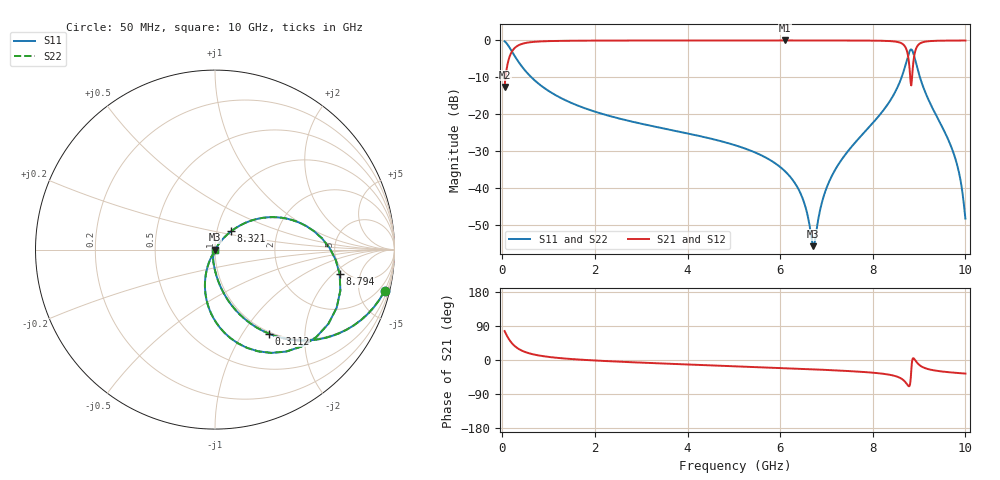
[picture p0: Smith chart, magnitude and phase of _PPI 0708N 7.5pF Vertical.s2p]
! S-Parameter data specifications (vertical orientation):
! Substrate: 40-mil Rogers 3003C, Substrate thickness, H=1.016mm, Dielectric constant, Er=3, Conductor thickness, T_mtl=0.043mm, Loss Tangent, Tand=0.003
! PCB Mounting Pad Footprint: Pad width, PadW=2.54mm , Pad length, PadL=0.51mm , Pad gap, PadG (edge-to-edge)=0.71mm , Reference planes=1.73mm apart
! Created Tue Jan 16 08:46:27 2018
# GHz S MA R 50
! 2 Port Network Data from SP1.SP block
! freq  magS11  angS11  magS21  angS21  magS12  angS12  magS22  angS22
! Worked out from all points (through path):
!   801 points, 50 MHz to 10 GHz, reference 50 ohm
!   highest |S21| = -0.02 dB at 6.107 GHz (marker M1); lowest = -12.6 dB at 50 MHz (marker M2)
!   group delay of S21, straight-line fit = 16 ps
!   lowest |S11| = -55.8 dB at 6.716 GHz (marker M3), VSWR 1.00, Z = 50.1 - j0.081 ohm
!   |S11| at or under -10 dB: 628.1 MHz to 8.622 GHz (7.994 GHz wide, 173 % of centre); 9.018 GHz to end of sweep
!   |S22| runs from -55.8 to -0.2 dB; largest |S21 - S12| = 0
!   S11 on the Smith chart (normalised r, x): 50 MHz: 0.97, -8.22; 311.2 MHz: 0.97, -1.32; 8.321 GHz: 1.17, +0.24; 8.794 GHz: 4.46, -2.45; 10 GHz: 1.00, -0.01
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0.05  0.9724 -13.7  0.2334 76.3  0.2334 76.3  0.9724 -13.7
0.1619375  0.7895 -38.5  0.6135 51.5  0.6135 51.5  0.7895 -38.5
0.3111875  0.5567 -57.3  0.8304 32.7  0.8304 32.7  0.5567 -57.3
0.7091875  0.2835 -76.1  0.9586 13.8  0.9586 13.8  0.2835 -76.1
1.716625  0.1245 -89.0  0.9916 0.7  0.9916 0.7  0.1245 -89.0
3.370812  0.06617 -98.1  0.9969 -8.8  0.9969 -8.8  0.06617 -98.1
5.025  0.03793 -104.9  0.998 -16.4  0.998 -16.4  0.03793 -104.9
6.107062  0.01677 -107.0  0.9983 -21.5  0.9983 -21.5  0.01677 -107.0
6.46775  0.007681 -102.2  0.9982 -23.4  0.9982 -23.4  0.007681 -102.2
6.691625  0.001853 -54.8  0.9981 -24.5  0.9981 -24.5  0.001853 -54.8
6.7165  0.001621 -29.9  0.9981 -24.7  0.9981 -24.7  0.001621 -29.9
6.927937  0.007269 50.3  0.9979 -25.8  0.9979 -25.8  0.007269 50.3
7.151813  0.01604 56.0  0.9976 -27.1  0.9976 -27.1  0.01604 56.0
8.320937  0.1355 48.6  0.9826 -38.0  0.9826 -38.0  0.1355 48.6
8.345812  0.1428 48.0  0.9809 -38.5  0.9809 -38.5  0.1428 48.0
8.681625  0.4094 25.8  0.8509 -55.3  0.8509 -55.3  0.4094 25.8
8.793563  0.7082 -11.1  0.4201 -68.5  0.4201 -68.5  0.7082 -11.1
8.880625  0.6555 -61.4  0.5342 4.7  0.5342 4.7  0.6555 -61.4
8.942813  0.4664 -83.5  0.7947 -5.2  0.7947 -5.2  0.4664 -83.5
9.029875  0.2997 -98.3  0.9174 -15.4  0.9174 -15.4  0.2997 -98.3
9.75125  0.02877 -115.4  0.9952 -33.5  0.9952 -33.5  0.02877 -115.4
10  0.003838 -59.9  0.9961 -35.8  0.9961 -35.8  0.003838 -59.9
